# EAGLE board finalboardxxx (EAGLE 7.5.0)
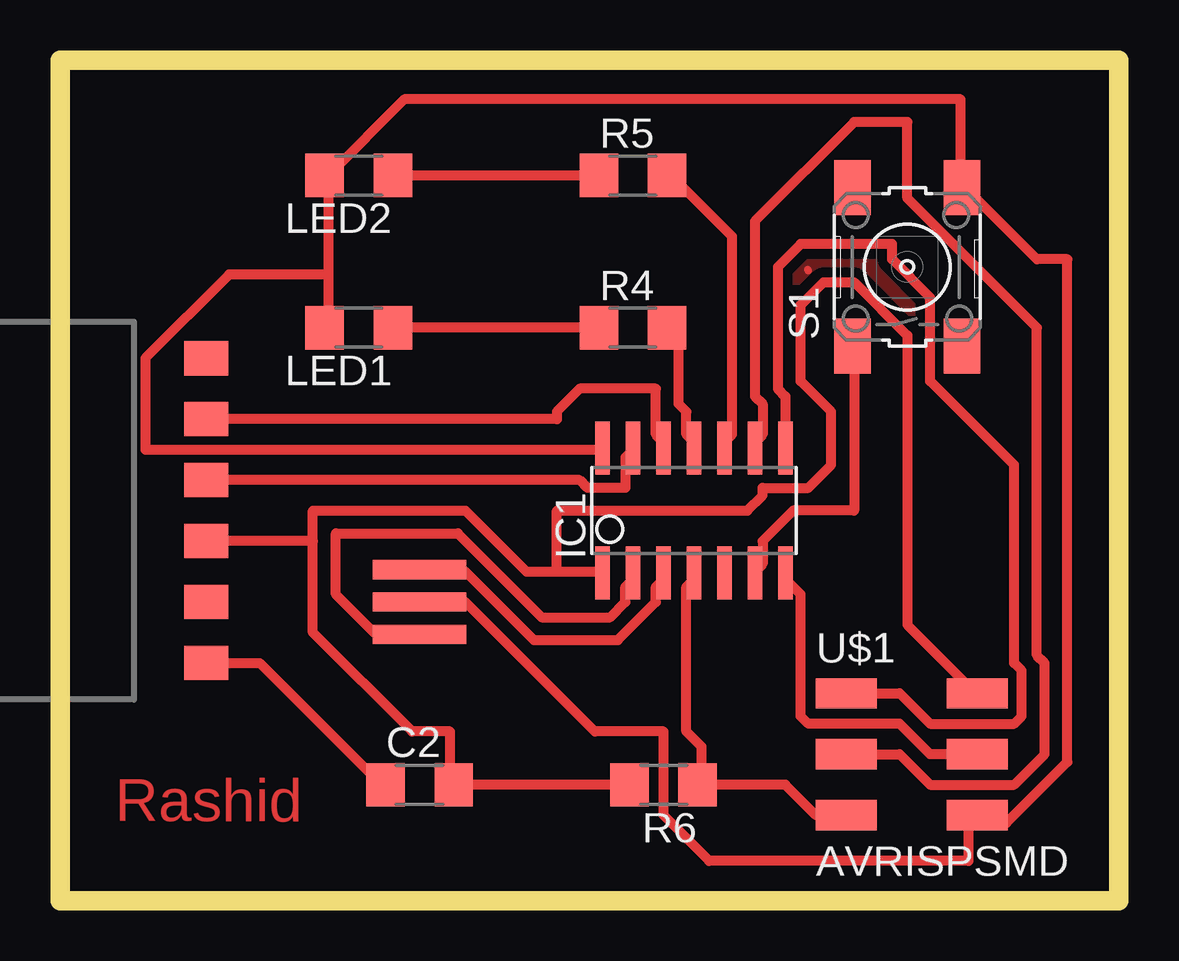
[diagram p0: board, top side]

Size 44.12 x 35.04 mm. Coordinates in mm from the lower left corner, seen from the top.
Outline: 0,0 44.12,0 44.12,35.04 0,35.04 0,0
Copper layers (1*16): Top 0.035mm / dielectric 1.5mm / Bottom 0.035mm
Design rules "default *": minimum track width 16mil, minimum drill 24mil, track to track 16mil, track to pad 12mil, pad to pad 8mil, via to via 8mil, smd to smd 8mil, copper to edge 40mil, drill to drill 8mil, minimum pad ring 10mil, minimum via ring 8mil, stop-mask expansion 4mil, vias tented up to drill 0mil, thermal gap 10mil
Net classes: 0 default: width 0.305 mm, drill 0.508 mm, clearance 0.254 mm

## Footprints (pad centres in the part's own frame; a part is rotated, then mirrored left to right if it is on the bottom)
1206 = smd 1.6 x 1.803: 1 -1.422,0; 2 1.422,0
SOIC14 = smd 0.61 x 2.21: 1 -3.81,-2.603; 2 -2.54,-2.603; 3 -1.27,-2.603; 4 0,-2.603; 5 1.27,-2.603; 6 2.54,-2.603; 7 3.81,-2.603; 8 3.81,2.603; 9 2.54,2.603; 10 1.27,2.603; 11 0,2.603; 12 -1.27,2.603; 13 -2.54,2.603; 14 -3.81,2.603
6MM_SWITCH = smd 2.286 x 1.524: 1 -3.302,2.286; 2 3.302,2.286; 3 -3.302,-2.286; 4 3.302,-2.286
2X03SMD = smd 2.54 x 1.27: 1 -2.54,2.54; 2 2.92,2.54; 3 -2.54,0; 4 2.92,0; 5 -2.54,-2.54; 6 2.92,-2.54
EFOBM = smd 0.8 x 3.9: 1 -1.35,0; 2 0,0; 3 1.35,0
SMH-106-XX-X-S = smd 1.422 x 1.829: 1 -6.35,0; 2 -3.81,0; 3 -1.27,0; 4 1.27,0; 5 3.81,0; 6 6.35,0

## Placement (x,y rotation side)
C2  11uf  [1206]  14.99,4.83 0 top
IC1  ATTINY44-SSU  [SOIC14]  26.42,16.26 0 top
LED1  [1206]  12.45,23.88 180 top
LED2  [1206]  12.45,30.23 180 top
R4  499  [1206]  23.88,23.88 0 top
R5  499  [1206]  23.88,30.23 0 top
R6  10K  [1206]  25.15,4.83 180 top
S1  [6MM_SWITCH]  35.31,26.42 90 top
U$1  AVRISPSMD  [2X03SMD]  35.31,6.1 0 top
U$2  RESONATOR 20MHZ  [EFOBM]  14.99,12.45 90 top
U$3  1X6.SMH.S  [SMH-106-XX-X-S]  6.1,16.26 90 top

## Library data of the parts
C2 LED1 LED2 R4-R6 U$1 = FAB_Hello
IC1 S1 U$2 = fab
U$3 = headers(.1in)(samtec)

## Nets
N$1: IC1.3 U$2.3
N$2: IC1.2 U$2.1
N$3: C2.1 U$3.1
N$4: IC1.4 R6.1 U$1.5
N$5: IC1.13 U$3.4
N$6: IC1.12 U$3.5
N$7: IC1.9 U$1.3
N$8: IC1.8 U$1.1
N$9: IC1.7 U$1.4
N$10: IC1.14 LED1.2 LED2.2 S1.4 U$1.6 U$2.2
N$11: IC1.11 R4.2
N$12: LED1.1 R4.1
N$13: LED2.1 R5.1
N$14: IC1.10 R5.2
N$15: IC1.6 S1.1
VCC: C2.2 IC1.1 R6.2 U$1.2 U$3.3

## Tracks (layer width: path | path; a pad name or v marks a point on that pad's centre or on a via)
GND
  Top 0.305: 31.18,26.26 31.16,26.3
  pour Top: -6.6,32.77 -6.6,2.29 41.66,2.29 41.66,32.77
N$1
  Top 0.406: IC1.3 25.15,13.4 24.83,13.08 24.83,12.45 23.24,10.86 19.75,10.86 16.89,13.72 14.99,13.72 U$2.3
N$2
  Top 0.406: IC1.2 23.88,13.4 23.56,13.08 23.56,12.45 22.92,11.81 20.07,11.81 16.57,15.3 11.49,15.3 11.49,12.76 13.08,11.18 14.99,11.18 U$2.1
N$3
  Top 0.406: U$3.1 8.32,9.91 13.4,4.83 C2.1
N$4
  Top 0.406: 26.73,4.83 30.23,4.83 31.5,3.56 U$1.5 | 26.73,4.83 26.73,6.41 26.1,7.05 26.1,13.08 26.42,13.4 IC1.4 | 26.73,4.83 R6.1
N$5
  Top 0.406: U$3.4 21.65,17.53 21.97,17.21 23.56,17.21 23.56,18.48 23.88,18.8 IC1.13
N$6
  Top 0.406: U$3.5 20.7,20.07 20.7,20.38 21.65,21.34 24.83,21.34 24.83,19.43 25.15,19.11 IC1.12
N$7
  Top 0.406: U$1.3 34.99,6.1 36.26,4.83 39.75,4.83 41.02,6.1 41.02,9.91 40.7,10.22 40.7,23.88 35.31,29.27 35.31,32.45 33.08,32.45 28.96,28.32 28.96,21.02 29.27,20.7 29.27,19.43 28.96,19.11 IC1.9
N$8
  Top 0.406: IC1.8 30.23,21.02 29.91,21.34 29.91,26.42 30.86,27.37 34.67,27.37 34.67,26.73 36.26,25.15 36.26,21.65 39.75,18.16 39.75,9.91 40.07,9.59 40.07,7.68 39.75,7.37 36.26,7.37 34.99,8.64 U$1.1
N$9
  Top 0.406: U$1.4 36.26,6.1 34.99,7.37 31.18,7.37 30.86,7.68 30.86,12.76 30.23,13.4 IC1.7
N$10
  Top 0.406: 11.18,30.23 11.18,26.1 | 11.18,26.1 11.18,23.88 LED1.2 | 11.18,26.1 7.05,26.1 3.56,22.61 3.56,18.8 22.61,18.8 IC1.14 | U$2.2 16.89,12.45 22.29,7.05 25.15,7.05 25.15,3.56 27.05,1.65 37.85,1.65 37.85,3.24 38.16,3.56 U$1.6 38.48,3.56 38.48,3.24 39.43,3.24 41.97,5.78 41.97,26.73 40.7,26.73 37.85,29.59 S1.4 37.53,29.91 37.53,33.4 14.35,33.4 11.18,30.23 | 11.18,30.23 LED2.2
N$11
  Top 0.406: R4.2 25.46,23.88 25.78,23.56 25.78,20.7 26.1,20.38 26.1,19.43 26.42,19.11 IC1.11
N$12
  Top 0.406: R4.1 LED1.1
N$13
  Top 0.406: R5.1 LED2.1
N$14
  Top 0.406: R5.2 25.46,30.23 28,27.69 28,19.43 27.69,19.11 IC1.10
N$15
  Top 0.406: IC1.6 28.96,13.72 29.27,14.03 29.27,14.99 30.54,16.26 33.08,16.26 33.08,22.92 S1.1
VCC
  Top 0.406: R6.2 C2.2 16.26,4.83 16.26,7.05 14.67,7.05 10.54,11.18 10.54,14.99 | 10.54,14.99 U$3.3 | 20.7,13.72 19.43,13.72 16.89,16.26 10.54,16.26 10.54,14.99 | 20.7,13.72 22.61,13.72 IC1.1 | 20.7,13.72 20.7,16.26 28.64,16.26 29.27,16.89 29.27,17.21 31.18,17.21 32.13,18.16 32.13,20.38 30.86,21.65 30.86,24.83 31.81,25.78 33.08,25.78 35.31,23.56 35.31,11.49 38.16,8.64 U$1.2

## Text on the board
Top: Rashid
